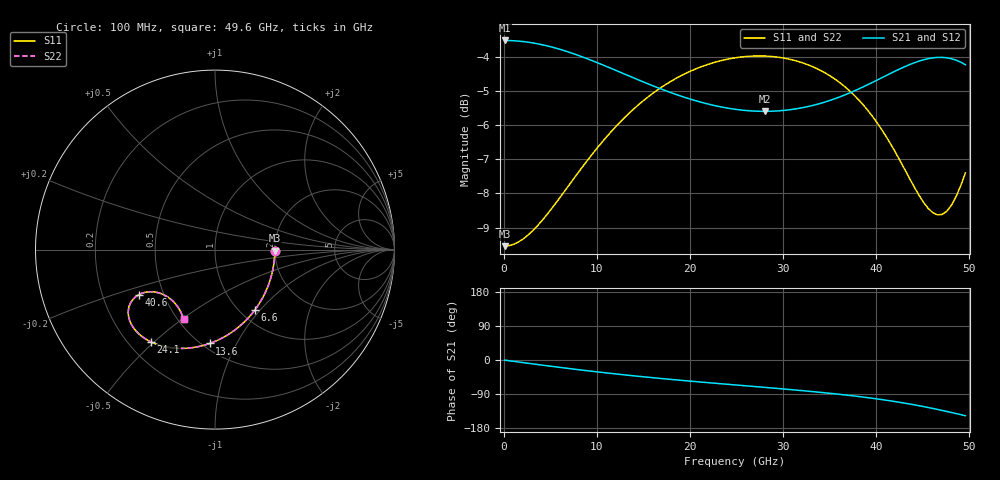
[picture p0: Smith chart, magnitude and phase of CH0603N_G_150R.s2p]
# GHz S RI R 150
! S-Parameters data
! Freq  reS11  imS11  reS21  imS21  reS12  imS12  reS22  imS22
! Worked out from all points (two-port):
!   100 points, 100 MHz to 49.6 GHz, reference 150 ohm
!   highest |S21| = -3.52 dB at 100 MHz (marker M1); lowest = -5.6 dB at 28.1 GHz (marker M2)
!   |S21| within 3 dB of the highest: start of sweep to end of sweep
!   lowest |S11| = -9.5 dB at 100 MHz (marker M3), VSWR 2.00, Z = 300 - j3.77 ohm
!   |S11| at or under -10 dB: nowhere
!   |S22| runs from -9.5 to -4.0 dB; largest |S21 - S12| = 0
!   S11 on the Smith chart (normalised r, x): 100 MHz: 2.00, -0.03; 6.6 GHz: 1.17, -0.94; 13.6 GHz: 0.54, -0.78; 24.1 GHz: 0.29, -0.49; 40.6 GHz: 0.36, -0.24; 49.6 GHz: 0.53, -0.51
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0.1  0.3333 -0.00558  0.6666 -0.00384  0.6666 -0.00384  0.3333 -0.00558
3.1  0.3074 -0.1693  0.6508 -0.1167  0.6508 -0.1167  0.3074 -0.1693
4.6  0.2776 -0.2447  0.6327 -0.1693  0.6327 -0.1693  0.2776 -0.2447
6.6  0.2237 -0.3342  0.5999 -0.2329  0.5999 -0.2329  0.2237 -0.3342
8.6  0.1578 -0.4084  0.5601 -0.2877  0.5601 -0.2877  0.1578 -0.4084
11.1  0.0658 -0.4781  0.5046 -0.3434  0.5046 -0.3434  0.0658 -0.4781
13.6  -0.0293 -0.5228  0.447 -0.3858  0.447 -0.3858  -0.0293 -0.5228
16.6  -0.139 -0.5478  0.3797 -0.4228  0.3797 -0.4228  -0.139 -0.5478
20.1  -0.2525 -0.5458  0.3067 -0.4527  0.3067 -0.4527  -0.2525 -0.5458
24.1  -0.3573 -0.5141  0.2308 -0.4778  0.2308 -0.4778  -0.3573 -0.5141
25.1  -0.379 -0.5026  0.2127 -0.4835  0.2127 -0.4835  -0.379 -0.5026
28.1  -0.4326 -0.4614  0.1589 -0.5004  0.1589 -0.5004  -0.4326 -0.4614
30.6  -0.4635 -0.4212  0.113 -0.5154  0.113 -0.5154  -0.4635 -0.4212
33.1  -0.4806 -0.3773  0.0632 -0.5314  0.0632 -0.5314  -0.4806 -0.3773
37.1  -0.474 -0.3048  -0.033 -0.5572  -0.033 -0.5572  -0.474 -0.3048
40.6  -0.4251 -0.2516  -0.1458 -0.5694  -0.1458 -0.5694  -0.4251 -0.2516
41.6  -0.4026 -0.2417  -0.1844 -0.5678  -0.1844 -0.5678  -0.4026 -0.2417
44.1  -0.3309 -0.237  -0.293 -0.5445  -0.293 -0.5445  -0.3309 -0.237
45.6  -0.2811 -0.2537  -0.3628 -0.5114  -0.3628 -0.5114  -0.2811 -0.2537
46.6  -0.2481 -0.2751  -0.4084 -0.4792  -0.4084 -0.4792  -0.2481 -0.2751
48.1  -0.2044 -0.3235  -0.4698 -0.4151  -0.4698 -0.4151  -0.2044 -0.3235
49.6  -0.1751 -0.3891  -0.5155 -0.3342  -0.5155 -0.3342  -0.1751 -0.3891
